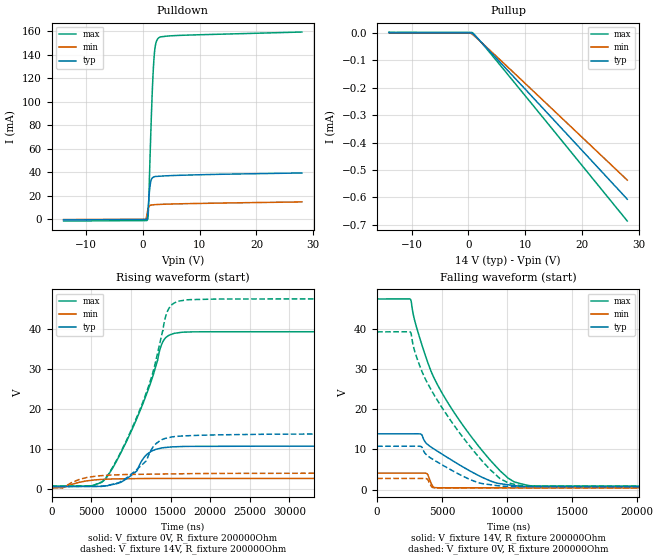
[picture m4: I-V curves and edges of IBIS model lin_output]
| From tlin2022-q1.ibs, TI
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|   lin_output Model
[Model]   lin_output
Model_type   Output
Polarity   Non-Inverting
Vmeas = 7
Vref = 0
Cref = 2pF
Rref = 100000
|   typ   min   max
C_comp   3.52891E-11   2.76465E-11   3.67824E-11
| Where Nom  PVT is Nominal Process, 14V, 27C
|   Fast PVT is Strong Process,  48V, -55C
|   Slow PVT is Weak Process,   4V, 165C
[Voltage Range]   14   4   48
|Junction Temperature
[Temperature Range]   27   165   -55
[Pullup Reference]   14   4   48
[Pulldown Reference]   -0   -0   0
[Power Clamp Reference]   14   4   48
[GND Clamp Reference]   0   0   0
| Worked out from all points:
|   slope of the pulldown table from 0 to 2.1 V, typ, clamps not added: 57.3 ohm
|   slope of the pullup table from 0 to 2.1 V, typ, clamps not added: 70.3 kohm
|   falling waveform, V_fixture 14V, R_fixture 200000Ohm: 20-80 % time 4us typ, 274ns min, 4.72us max; typ from 13.9 V to 0.714 V
|   rising waveform, V_fixture 0V, R_fixture 200000Ohm: 20-80 % time 2.54us typ, 3.06us min, 4.7us max; typ from 0.706 V to 10.8 V
|   rising waveform, V_fixture 14V, R_fixture 200000Ohm: 20-80 % time 3.32us typ, 3.75us min, 4.91us max; typ from 0.714 V to 13.9 V
|   falling waveform, V_fixture 0V, R_fixture 200000Ohm: 20-80 % time 3.24us typ, 227ns min, 4.52us max; typ from 10.8 V to 0.706 V
[Pulldown]
|   Voltage   I(typ)   I(min)   I(max)
-14V      -605.9uA   -340uA     -1.551mA
238mV     -286.7uA   -59.26uA   -1.187mA
532mV     -278.1uA   589.6uA    -1.179mA
784mV     1.64mA     6.469mA    -489.8uA
868mV     6.335mA    8.362mA    927.5uA
952mV     12.21mA    9.778mA    7.793mA
1.288V    29.99mA    11.85mA    60.72mA
1.624V    35.04mA    12.19mA    107.8mA
1.876V    35.95mA    12.31mA    132.9mA
2.212V    36.47mA    12.42mA    148.8mA
2.8V      36.56mA    12.57mA    154.6mA
28V       39.37mA    14.71mA    159.4mA
[Pullup]
|   Voltage   I(typ)   I(min)   I(max)
-14V      1.413uA    828.1nA    3.686uA
280mV     80.68nA    -512.6nA   2.277uA
742mV     -1.698uA   -5.465uA   443.9nA
2.254V    -33.13uA   -33.45uA   -33.96uA
5.32V     -100.7uA   -92.63uA   -110.3uA
28V       -606.3uA   -536.7uA   -686uA
[Ramp]
R_load = 200000
|   typ   min   max
dV/dt_r   6.04162/2.54047e-06   1.40453/3.01133e-06   23.0598/4.70296e-06
dV/dt_f   7.88762/4.00556e-06   2.19955/2.7349e-07   27.9616/4.72345e-06
[Falling Waveform]
V_fixture = 14V
V_fixture_min = 4V
V_fixture_max = 48V
R_fixture = 200000Ohm
C_fixture = 0F
|   Time   V(typ)   V(min)   V(max)
0s        13.86V     4.089V     47.44V
2.568us   13.87V     4.096V     47.36V
3.417us   13.71V     4.098V     36.34V
4.012us   10.9V      2.775V     30.63V
4.424us   9.997V     470.6mV    27.5V
5.893us   7.015V     426.5mV    19.35V
9.457us   1.462V     426.4mV    4.68V
10.53us   989.4mV    426.4mV    1.929V
12.01us   744.7mV    426.4mV    891.8mV
250us     713.9mV    422.8mV    840.7mV
[Rising Waveform]
V_fixture = 0V
V_fixture_min = 0V
V_fixture_max = 0V
R_fixture = 200000Ohm
C_fixture = 0F
|   Time   V(typ)   V(min)   V(max)
0s        705.7mV    415.5mV    826.3mV
5.149us   749.5mV    2.302V     926.4mV
6.767us   862.8mV    2.538V     2.602V
8.238us   1.464V     2.636V     7.266V
10.53us   4.276V     2.688V     16.7V
12.02us   8.741V     2.722V     24V
14.02us   10.37V     2.731V     36.75V
14.9us    10.54V     2.731V     38.48V
16.42us   10.68V     2.731V     39.13V
250us     10.78V     2.756V     39.26V
[Rising Waveform]
V_fixture = 14V
V_fixture_min = 4V
V_fixture_max = 48V
R_fixture = 200000Ohm
C_fixture = 0F
|   Time   V(typ)   V(min)   V(max)
0s        713.9mV    422.8mV    840.7mV
5.149us   763.1mV    3.181V     962.7mV
6.97us    964.8mV    3.527V     3.251V
9.457us   2.898V     3.72V      12.3V
12.01us   7.436V     3.788V     24.49V
13.17us   11.42V     3.818V     32.31V
14.66us   12.85V     3.857V     44.61V
15.48us   13.15V     3.879V     46.44V
17us      13.36V     3.918V     47.19V
250us     13.86V     4.089V     47.44V
[Falling Waveform]
|Gnd
V_fixture = 0V
V_fixture_min = 0V
V_fixture_max = 0V
R_fixture = 200000Ohm
C_fixture = 0F
|   Time   V(typ)   V(min)   V(max)
0s        10.78V     2.756V     39.26V
2.568us   10.79V     2.763V     39.18V
2.941us   10.79V     2.764V     33.96V
3.417us   10.65V     2.765V     29.69V
3.72us    8.922V     2.74V      27.49V
4.295us   7.512V     482.2mV    24.08V
6.318us   3.793V     418.1mV    14.23V
9.457us   889.2mV    418mV      2.725V
11.34us   726.9mV    418mV      873.5mV
250us     705.7mV    415.5mV    826.3mV
